| IBIS file imx8qx_21x21_v204.ibs generated by Viper version: 2017.04.12
[IBIS Ver]   6.0
[Comment Char] |_char
[File name]   imx8qxp_21x21_v204.ibs
[File Rev]   2.04
[Date]   Nov 13,2019
[Source]   NXP Viper 2017.04.12
[Notes]
   Warning 'pullup_ref' Exceeds 15 characters: VDD_PCIE_LDO_1P0_CAP was cut to VDD_PCIE_LDO_1P
   Warning 'pullup_ref' Exceeds 15 characters: VDD_PCIE_DIG_1P8_3P3 was cut to VDD_PCIE_DIG_1P
   Warning 'pullup_ref' Exceeds 15 characters: VDD_USB_SS3_LDO_1P0_CAP was cut to VDD_USB_SS3_LDO
   Warning 'pullup_ref' Exceeds 15 characters: VDD_EMMC0_1P8_3P3 was cut to VDD_EMMC0_1P8_3
   Warning 'pullup_ref' Exceeds 15 characters: VDD_EMMC0_VSELECT_1P8_3P3 was cut to VDD_EMMC0_VSELE
   Warning 'pullup_ref' Exceeds 15 characters: VDD_USDHC1_VSELECT_1P8_3P3 was cut to VDD_USDHC1_VSEL
   Warning 'pullup_ref' Exceeds 15 characters: VDD_USDHC1_1P8_3P3 was cut to VDD_USDHC1_1P8_
   Warning 'pullup_ref' Exceeds 15 characters: VDD_ENET0_VSELECT_1P8_2P5_3P3 was cut to VDD_ENET0_VSELE
   Warning 'pullup_ref' Exceeds 15 characters: VDD_ENET0_1P8_2P5_3P3 was cut to VDD_ENET0_1P8_2
   Warning 'pullup_ref' Exceeds 15 characters: VDD_ENET_MDIO_1P8_3P3 was cut to VDD_ENET_MDIO_1
   Warning 'pullup_ref' Exceeds 15 characters: VDD_ESAI_SPDIF_1P8_2P5_3P3 was cut to VDD_ESAI_SPDIF_
   Warning 'pullup_ref' Exceeds 15 characters: VDD_SPI_MCLK_UART_1P8_3P3 was cut to VDD_SPI_MCLK_UA
   Warning 'pullup_ref' Exceeds 15 characters: PCIE0_PHY_PLL_REF_RETURN was cut to PCIE0_PHY_PLL_R
   Warning 'pullup_ref' Exceeds 15 characters: VDD_SPI_SAI_1P8_3P3 was cut to VDD_SPI_SAI_1P8
   Warning 'pullup_ref' Exceeds 15 characters: VDD_PCIE_LDO_1P0_CAP was cut to VDD_PCIE_LDO_1P
   Warning 'pullup_ref' Exceeds 15 characters: VDD_CAN_UART_1P8_3P3 was cut to VDD_CAN_UART_1P
   Warning 'pullup_ref' Exceeds 15 characters: VDD_MIPI_DSI_DIG_1P8_3P3 was cut to VDD_MIPI_DSI_DI
   Warning 'pullup_ref' Exceeds 15 characters: VDD_TMPR_CSI_1P8_3P3 was cut to VDD_TMPR_CSI_1P
   Warning 'pullup_ref' Exceeds 15 characters: VDD_QSPI0B_1P8_3P3 was cut to VDD_QSPI0B_1P8_
   Warning 'pulldown_ref' Exceeds 15 characters: VDD_MIPI_CSI_DIG_1P8 was cut to  VDD_MIPI_CSI_DI
   Warning 'pullup_ref' Exceeds 15 characters: VDD_QSPI0A_1P8_3P3 was cut to VDD_QSPI0A_1P8_
   Warning 'pulldown_ref' Exceeds 15 characters: VDD_SNVS_LDO_1P8_CAP was cut to VDD_SNVS_LDO_1P
[Disclaimer] IMPORTANT NOTICE
  This information is provided on an AS IS basis and without warranty.
  IN NO EVENT SHALL NXP BE LIABLE FOR INCIDENTAL OR CONSEQUENTIAL
  DAMAGES ARISING FROM USE OF THIS INFORMATION. THIS DISCLAIMER OF
  WARRANTY EXTENDS TO THE USER OF THE INFORMATION, AND TO THEIR CUSTOMERS
  OR USERS OF PRODUCTS  AND IS IN LIEU OF ALL WARRANTIES WHETHER EXPRESS,
  IMPLIED, OR STATUTORY, INCLUDING IMPLIED WARRANTIES OF MERCHANTABILITY
  OR FITNESS FOR PARTICULAR PURPOSE.
  NXP does not represent or warrant that the information furnished
  hereunder is free of infringement of any third party patents,
  copyrights, trade secrets, or other intellectual property rights.
  NXP does not represent or warrant that the information is free of
  defect, or that it meets any particular standard, requirements or need
  of the user of the infomation or their customers.
  NXP reserves the right to change the information in this file
  without notice.
   http://www.nxp.com
[Copyright]   (C) Copyright NXP 2006 - 2019, All Rights Reserved.
|   imx8qxp_21x21
[Component] imx8qxp_21x21_v204
[Manufacturer] NXP
[Package]
|   typ   min   max
R_pkg   0.40366   0.037637   0.82546
L_pkg   2.483e-9   4.73e-10   4.759e-9
C_pkg   1.224e-12   7.498e-13   3.887e-12
[Pin]   Signal_name   model_name   R_pin   L_pin   C_pin
AA15   VDD_A35   POWER   0.00219   4.708e-11   1.478e-11
AA17   VDD_A35   POWER   0.00219   4.708e-11   1.478e-11
AA19   VDD_A35   POWER   0.00219   4.708e-11   1.478e-11
AB16   VDD_A35   POWER   0.00219   4.708e-11   1.478e-11
AB18   VDD_A35   POWER   0.00219   4.708e-11   1.478e-11
AB20   VDD_A35   POWER   0.00219   4.708e-11   1.478e-11
V28   VDD_ADC_1P8   POWER   0.04684   4.968e-10   1.587e-12
W25   VDD_ADC_DIG_1P8   POWER   0.02408   3.35e-10   7.513e-13
M14   VDD_ANA0_1P8   POWER   0.02045   2.873e-10   3.689e-12
AB24   VDD_ANA1_1P8   POWER   0.01003   1.805e-10   3.242e-12
Y24   VDD_CAN_UART_1P8_3P3   POWER   0.02207   3.294e-10   7.089e-13
AE23   VDD_CSI_1P8_3P3   POWER   0.0291   4.307e-10   1.073e-12
AC9   VDD_DDR_PLL_1P8   POWER   0.03235   4.677e-10   3.486e-12
AA9   VDD_DDR_VDDQ   POWER   0.00256   3.19e-11   2.867e-11
AA11   VDD_DDR_VDDQ   POWER   0.00256   3.19e-11   2.867e-11
AC11   VDD_DDR_VDDQ   POWER   0.00256   3.19e-11   2.867e-11
AD12   VDD_DDR_VDDQ   POWER   0.00256   3.19e-11   2.867e-11
AE11   VDD_DDR_VDDQ   POWER   0.00256   3.19e-11   2.867e-11
M12   VDD_DDR_VDDQ   POWER   0.00256   3.19e-11   2.867e-11
N9   VDD_DDR_VDDQ   POWER   0.00256   3.19e-11   2.867e-11
N11   VDD_DDR_VDDQ   POWER   0.00256   3.19e-11   2.867e-11
R7   VDD_DDR_VDDQ   POWER   0.00256   3.19e-11   2.867e-11
R11   VDD_DDR_VDDQ   POWER   0.00256   3.19e-11   2.867e-11
T12   VDD_DDR_VDDQ   POWER   0.00256   3.19e-11   2.867e-11
U11   VDD_DDR_VDDQ   POWER   0.00256   3.19e-11   2.867e-11
W11   VDD_DDR_VDDQ   POWER   0.00256   3.19e-11   2.867e-11
Y12   VDD_DDR_VDDQ   POWER   0.00256   3.19e-11   2.867e-11
L19   VDD_EMMC0_1P8_3P3   POWER   0.02931   4.406e-10   9.586e-13
M20   VDD_EMMC0_VSELECT_1P8_3P3   POWER   0.0289   4.327e-10   6.925e-13
M24   VDD_ENET0_1P8_2P5_3P3   POWER   0.02439   3.623e-10   7.403e-13
L23   VDD_ENET0_VSELECT_1P8_2P5_3P3   POWER   0.02814   4.601e-10   1.125e-12
L25   VDD_ENET_MDIO_1P8_3P3   POWER   0.0233   3.037e-10   9.528e-13
N25   VDD_ESAI_SPDIF_1P8_2P5_3P3   POWER   0.01663   2.138e-10   1.247e-12
N23   VDD_GPU   POWER   0.00187   3.523e-11   2.181e-11
P20   VDD_GPU   POWER   0.00187   3.523e-11   2.181e-11
P22   VDD_GPU   POWER   0.00187   3.523e-11   2.181e-11
R21   VDD_GPU   POWER   0.00187   3.523e-11   2.181e-11
T22   VDD_GPU   POWER   0.00187   3.523e-11   2.181e-11
U23   VDD_GPU   POWER   0.00187   3.523e-11   2.181e-11
V20   VDD_GPU   POWER   0.00187   3.523e-11   2.181e-11
W21   VDD_GPU   POWER   0.00187   3.523e-11   2.181e-11
AA23   VDD_MAIN   POWER   0.00038   7.636e-12   1.284e-10
AB12   VDD_MAIN   POWER   0.00038   7.636e-12   1.284e-10
AC13   VDD_MAIN   POWER   0.00038   7.636e-12   1.284e-10
AC17   VDD_MAIN   POWER   0.00038   7.636e-12   1.284e-10
AC21   VDD_MAIN   POWER   0.00038   7.636e-12   1.284e-10
AD14   VDD_MAIN   POWER   0.00038   7.636e-12   1.284e-10
AD22   VDD_MAIN   POWER   0.00038   7.636e-12   1.284e-10
N15   VDD_MAIN   POWER   0.00038   7.636e-12   1.284e-10
N19   VDD_MAIN   POWER   0.00038   7.636e-12   1.284e-10
P12   VDD_MAIN   POWER   0.00038   7.636e-12   1.284e-10
P16   VDD_MAIN   POWER   0.00038   7.636e-12   1.284e-10
P24   VDD_MAIN   POWER   0.00038   7.636e-12   1.284e-10
R13   VDD_MAIN   POWER   0.00038   7.636e-12   1.284e-10
R17   VDD_MAIN   POWER   0.00038   7.636e-12   1.284e-10
T14   VDD_MAIN   POWER   0.00038   7.636e-12   1.284e-10
T18   VDD_MAIN   POWER   0.00038   7.636e-12   1.284e-10
U15   VDD_MAIN   POWER   0.00038   7.636e-12   1.284e-10
U19   VDD_MAIN   POWER   0.00038   7.636e-12   1.284e-10
V12   VDD_MAIN   POWER   0.00038   7.636e-12   1.284e-10
V16   VDD_MAIN   POWER   0.00038   7.636e-12   1.284e-10
V24   VDD_MAIN   POWER   0.00038   7.636e-12   1.284e-10
W13   VDD_MAIN   POWER   0.00038   7.636e-12   1.284e-10
W17   VDD_MAIN   POWER   0.00038   7.636e-12   1.284e-10
Y14   VDD_MAIN   POWER   0.00038   7.636e-12   1.284e-10
Y18   VDD_MAIN   POWER   0.00038   7.636e-12   1.284e-10
Y22   VDD_MAIN   POWER   0.00038   7.636e-12   1.284e-10
AD18   VDD_MIPI_1P0   POWER   0.00784   1.178e-10   4.481e-12
AE19   VDD_MIPI_1P0   POWER   0.00784   1.178e-10   4.481e-12
AD16   VDD_MIPI_1P8   POWER   0.00846   1.296e-10   3.255e-12
AE17   VDD_MIPI_1P8   POWER   0.00846   1.296e-10   3.255e-12
AE21   VDD_MIPI_CSI_DIG_1P8   POWER   0.02051   3.356e-10   8.748e-13
AA25   VDD_MIPI_DSI_DIG_1P8_3P3   POWER   0.0223   3.942e-10   7.725e-13
G13   VDD_PCIE_1P8   POWER   0.05261   4.939e-10   2.52e-12
L11   VDD_PCIE_DIG_1P8_3P3   POWER   0.02609   3.742e-10   9.301e-13
L13   VDD_PCIE_LDO_1P0_CAP   POWER   0.02621   2.855e-10   1.291e-12
AE15   VDD_QSPI0A_1P8_3P3   POWER   0.02715   4.596e-10   9.514e-13
AE13   VDD_QSPI0B_1P8_3P3   POWER   0.02591   4.435e-10   9.193e-13
AC25   VDD_SNVS_4P2   POWER   0.04094   4.39e-10   1.24e-12
AE25   VDD_SNVS_LDO_1P8_CAP   POWER   0.02861   4.218e-10   9.798e-13
R25   VDD_SPI_MCLK_UART_1P8_3P3   POWER   0.02101   3.863e-10   9.493e-13
U25   VDD_SPI_SAI_1P8_3P3   POWER   0.01791   3.169e-10   1.118e-12
AD24   VDD_TMPR_CSI_1P8_3P3   POWER   0.02854   4.826e-10   6.671e-13
M18   VDD_USB_1P8   POWER   0.01867   2.529e-10   1.459e-12
L15   VDD_USB_3P3   POWER   0.01456   2.231e-10   2.366e-12
L17   VDD_USB_OTG_1P0   POWER   0.02825   3.838e-10   7.015e-13
M16   VDD_USB_SS3_LDO_1P0_CAP   POWER   0.02218   3.197e-10   1.184e-12
M22   VDD_USDHC1_1P8_3P3   POWER   0.02734   4.514e-10   8.749e-13
L21   VDD_USDHC1_VSELECT_1P8_3P3   POWER   0.02938   4.213e-10   8.418e-13
U35   ADC_IN0   CSF_1V8_FCGPIO   0.42651   2.631e-9   1.261e-12
U33   ADC_IN1   CSF_1V8_FCGPIO   0.36525   2.261e-9   1.117e-12
V32   ADC_IN2   CSF_1V8_FCGPIO   0.31185   1.955e-9   1.06e-12
V30   ADC_IN3   CSF_1V8_FCGPIO   0.27174   1.778e-9   9.234e-13
W29   ADC_IN4   CSF_1V8_FCGPIO   0.22361   1.51e-9   9.133e-13
V34   ADC_IN5   CSF_1V8_FCGPIO   0.38226   2.352e-9   1.137e-12
U29   ADC_VREFH   POWER   0.16541   1.336e-9   1.06e-12
U31   ADC_VREFL   GND   0.16331   1.278e-9   1.113e-12
AK34   ANA_TEST_OUT_N   NC   0.55674   3.419e-9   1.479e-12
AL35   ANA_TEST_OUT_P   NC   0.55489   3.454e-9   1.49e-12
AK28   CSI_D00   IO_20UM_RES_ANAF   0.30952   1.939e-9   1.008e-12
AL29   CSI_D01   IO_20UM_RES_ANAF   0.37926   2.374e-9   1.138e-12
AP30   CSI_D02   IO_20UM_RES_ANAF   0.50676   3.048e-9   1.397e-12
AJ27   CSI_D03   IO_20UM_RES_ANAF   0.26395   1.704e-9   9.425e-13
AN29   CSI_D04   IO_20UM_RES_ANAF   0.44676   2.71e-9   1.306e-12
AM30   CSI_D05   IO_20UM_RES_ANAF   0.49033   2.894e-9   1.387e-12
AJ25   CSI_D06   IO_20UM_RES_ANAF   0.23567   1.526e-9   9.239e-13
AM28   CSI_D07   IO_20UM_RES_ANAF   0.44578   2.645e-9   1.28e-12
AP28   CSI_EN   3V3SF_1V8_3V3_FCGPIO   0.51053   3.054e-9   1.418e-12
AR29   CSI_HSYNC   IO_20UM_RES_ANAF   0.50745   3.087e-9   1.399e-12
AM26   CSI_MCLK   3V3SF_1V8_3V3_FCGPIO   0.3713   2.281e-9   1.19e-12
AK26   CSI_PCLK   3V3SF_1V8_3V3_FCGPIO   0.32277   2.042e-9   1.037e-12
AR27   CSI_RESET   3V3SF_1V8_3V3_FCGPIO   0.48863   3.001e-9   1.374e-12
AL27   CSI_VSYNC   IO_20UM_RES_ANAF   0.36588   2.261e-9   1.126e-12
AB8   DDR_ATO   NC   0.34374   2.177e-9   9.917e-13
Y6   DDR_CK0_N   PCK_PAD   0.32055   2.016e-9   1.025e-12
W5   DDR_CK0_P   PCK_PAD   0.30751   1.935e-9   1.05e-12
N5   DDR_CK1_N   PCK_PAD   0.34912   2.078e-9   1.033e-12
P6   DDR_CK1_P   PCK_PAD   0.3404   2.05e-9   1.067e-12
W1   DDR_DCF00   PCKE_PAD   0.4081   2.466e-9   1.201e-12
U3   DDR_DCF01   PCKE_PAD   0.39573   2.365e-9   1.079e-12
U1   DDR_DCF03   PCKE_PAD   0.41209   2.476e-9   1.189e-12
U7   DDR_DCF04   PCKE_PAD   0.26915   1.653e-9   8.978e-13
U5   DDR_DCF05   PCKE_PAD   0.28802   1.762e-9   9.477e-13
T2   DDR_DCF07   PCKE_PAD   0.38159   2.286e-9   1.123e-12
AB4   DDR_DCF08   PCKE_PAD   0.33535   2.032e-9   1.075e-12
AB6   DDR_DCF09   PCKE_PAD   0.31122   1.881e-9   1.054e-12
AC5   DDR_DCF10   PCKE_PAD   0.42271   2.539e-9   1.134e-12
W3   DDR_DCF11   PCKE_PAD   0.39581   2.382e-9   1.165e-12
Y8   DDR_DCF12   PCKE_PAD   0.26258   1.59e-9   8.647e-13
Y2   DDR_DCF14   PCKE_PAD   0.43988   2.601e-9   1.26e-12
Y4   DDR_DCF15   PCKE_PAD   0.39283   2.343e-9   1.098e-12
W7   DDR_DCF16   PCKE_PAD   0.22506   1.423e-9   8.936e-13
N3   DDR_DCF17   PCKE_PAD   0.40043   2.368e-9   1.158e-12
L1   DDR_DCF18   PCKE_PAD   0.54939   3.23e-9   1.358e-12
N1   DDR_DCF19   PCKE_PAD   0.47195   2.811e-9   1.296e-12
P4   DDR_DCF20   PCKE_PAD   0.38159   2.233e-9   1.089e-12
T8   DDR_DCF21   PCKE_PAD   0.22786   1.416e-9   8.827e-13
P2   DDR_DCF22   PCKE_PAD   0.44786   2.591e-9   1.196e-12
T4   DDR_DCF23   PCKE_PAD   0.30475   1.872e-9   1.03e-12
T6   DDR_DCF24   PCKE_PAD   0.30086   1.802e-9   9.477e-13
K8   DDR_DCF25   PCKE_PAD   0.37204   2.249e-9   1.113e-12
L7   DDR_DCF26   PCKE_PAD   0.31491   2.008e-9   9.604e-13
K4   DDR_DCF27   PCKE_PAD   0.412   2.421e-9   1.164e-12
K6   DDR_DCF28   PCKE_PAD   0.39245   2.305e-9   1.103e-12
K2   DDR_DCF29   PCKE_PAD   0.46305   2.734e-9   1.263e-12
N7   DDR_DCF30   PCKE_PAD   0.21434   1.379e-9   8.174e-13
L5   DDR_DCF31   PCKE_PAD   0.42725   2.616e-9   1.143e-12
L3   DDR_DCF32   PCKE_PAD   0.41678   2.499e-9   1.169e-12
P8   DDR_DCF33   PCKE_PAD   0.18645   1.263e-9   7.498e-13
AJ7   DDR_DM0   PDDRIO_PAD   0.38383   2.275e-9   1.142e-12
AF4   DDR_DM1   PDDRIO_PAD   0.40315   2.392e-9   1.179e-12
D4   DDR_DM2   PDDRIO_PAD   0.53266   3.078e-9   1.418e-12
E1   DDR_DM3   PDDRIO_PAD   0.74086   4.27e-9   1.815e-12
AP6   DDR_DM4   PDDRIO_PAD   0.48564   2.866e-9   1.328e-12
AF6   DDR_DQ00   PDDRIO_PAD   0.34789   2.063e-9   9.964e-13
AE5   DDR_DQ01   PDDRIO_PAD   0.30627   1.861e-9   1.026e-12
AH8   DDR_DQ02   PDDRIO_PAD   0.38806   2.264e-9   1.109e-12
AF8   DDR_DQ03   PDDRIO_PAD   0.30103   1.788e-9   1.013e-12
AM4   DDR_DQ04   PDDRIO_PAD   0.53729   3.098e-9   1.447e-12
AM6   DDR_DQ05   PDDRIO_PAD   0.55824   3.2e-9   1.443e-12
AL5   DDR_DQ06   PDDRIO_PAD   0.47532   2.794e-9   1.344e-12
AL7   DDR_DQ07   PDDRIO_PAD   0.50156   2.927e-9   1.333e-12
AJ1   DDR_DQ08   PDDRIO_PAD   0.55986   3.265e-9   1.485e-12
AJ3   DDR_DQ09   PDDRIO_PAD   0.51931   2.978e-9   1.364e-12
AH2   DDR_DQ10   PDDRIO_PAD   0.52291   3.031e-9   1.394e-12
AH4   DDR_DQ11   PDDRIO_PAD   0.48438   2.816e-9   1.311e-12
AC3   DDR_DQ12   PDDRIO_PAD   0.39385   2.334e-9   1.15e-12
AE3   DDR_DQ13   PDDRIO_PAD   0.44737   2.593e-9   1.227e-12
AB2   DDR_DQ14   PDDRIO_PAD   0.43448   2.589e-9   1.216e-12
AC1   DDR_DQ15   PDDRIO_PAD   0.50595   3.028e-9   1.287e-12
B6   DDR_DQ16   PDDRIO_PAD   0.60749   3.574e-9   1.522e-12
E9   DDR_DQ17   PDDRIO_PAD   0.50742   3.111e-9   1.313e-12
E7   DDR_DQ18   PDDRIO_PAD   0.4559   2.689e-9   1.295e-12
D8   DDR_DQ19   PDDRIO_PAD   0.54325   3.262e-9   1.355e-12
G7   DDR_DQ20   PDDRIO_PAD   0.46743   2.712e-9   1.304e-12
H8   DDR_DQ21   PDDRIO_PAD   0.50906   2.936e-9   1.288e-12
H6   DDR_DQ22   PDDRIO_PAD   0.4057   2.436e-9   1.192e-12
G5   DDR_DQ23   PDDRIO_PAD   0.45898   2.662e-9   1.251e-12
H2   DDR_DQ24   PDDRIO_PAD   0.77451   4.461e-9   1.879e-12
H4   DDR_DQ25   PDDRIO_PAD   0.7738   4.561e-9   1.785e-12
G3   DDR_DQ26   PDDRIO_PAD   0.73029   4.212e-9   1.787e-12
G1   DDR_DQ27   PDDRIO_PAD   0.82546   4.759e-9   1.895e-12
A7   DDR_DQ28   PDDRIO_PAD   0.5151   3.062e-9   1.35e-12
B4   DDR_DQ29   PDDRIO_PAD   0.58541   3.377e-9   1.536e-12
B2   DDR_DQ30   PDDRIO_PAD   0.64864   3.755e-9   1.64e-12
A5   DDR_DQ31   PDDRIO_PAD   0.55394   3.304e-9   1.492e-12
AL1   DDR_DQ32   PDDRIO_PAD   0.69902   3.996e-9   1.723e-12
AM2   DDR_DQ33   PDDRIO_PAD   0.68978   3.899e-9   1.65e-12
AL3   DDR_DQ34   PDDRIO_PAD   0.60728   3.501e-9   1.582e-12
AP2   DDR_DQ35   PDDRIO_PAD   0.73516   4.145e-9   1.724e-12
AP8   DDR_DQ36   PDDRIO_PAD   0.45415   2.678e-9   1.278e-12
AP10   DDR_DQ37   PDDRIO_PAD   0.49344   2.899e-9   1.314e-12
AR9   DDR_DQ38   PDDRIO_PAD   0.50308   2.973e-9   1.338e-12
AR7   DDR_DQ39   PDDRIO_PAD   0.48449   2.912e-9   1.388e-12
AH6   DDR_DQS0_N   PDQS_PAD   0.47602   2.752e-9   1.322e-12
AJ5   DDR_DQS0_P   PDQS_PAD   0.48689   2.789e-9   1.302e-12
AE1   DDR_DQS1_N   PDQS_PAD   0.53539   3.09e-9   1.4e-12
AF2   DDR_DQS1_P   PDQS_PAD   0.52472   3.013e-9   1.398e-12
E5   DDR_DQS2_N   PDQS_PAD   0.54029   3.111e-9   1.395e-12
D6   DDR_DQS2_P   PDQS_PAD   0.54822   3.239e-9   1.375e-12
E3   DDR_DQS3_N   PDQS_PAD   0.75887   4.285e-9   1.793e-12
D2   DDR_DQS3_P   PDQS_PAD   0.74586   4.218e-9   1.843e-12
AR5   DDR_DQS4_N   PDQS_PAD   0.62598   3.596e-9   1.508e-12
AP4   DDR_DQS4_P   PDQS_PAD   0.61626   3.503e-9   1.593e-12
AC7   DDR_DTO0   PDDRIO_PAD   0.37637   2.321e-9   1.141e-12
AE7   DDR_DTO1   PDDRIO_PAD   0.40575   2.477e-9   1.172e-12
AD8   DDR_VREF   POWER   0.037637   4.73e-10   3.887e-12
G9   DDR_ZQ   NC   0.47928   3.163e-9   2.009e-12
G19   EMMC0_CLK   3V3SF_1V8_3V3_FCGPIO   0.24299   1.577e-9   9.178e-13
D20   EMMC0_CMD   3V3SF_1V8_3V3_FCGPIO   0.35749   2.183e-9   1.114e-12
C21   EMMC0_DATA0   3V3SF_1V8_3V3_FCGPIO   0.40233   2.452e-9   1.222e-12
A21   EMMC0_DATA1   3V3SF_1V8_3V3_FCGPIO   0.43389   2.669e-9   1.273e-12
E21   EMMC0_DATA2   3V3SF_1V8_3V3_FCGPIO   0.34577   2.14e-9   1.047e-12
H20   EMMC0_DATA3   3V3SF_1V8_3V3_FCGPIO   0.19693   1.326e-9   8.274e-13
B22   EMMC0_DATA4   3V3SF_1V8_3V3_FCGPIO   0.40922   2.519e-9   1.201e-12
G21   EMMC0_DATA5   3V3SF_1V8_3V3_FCGPIO   0.2411   1.561e-9   8.981e-13
A23   EMMC0_DATA6   3V3SF_1V8_3V3_FCGPIO   0.47648   2.905e-9   1.346e-12
D22   EMMC0_DATA7   3V3SF_1V8_3V3_FCGPIO   0.38392   2.379e-9   1.207e-12
H22   EMMC0_RESET_B   3V3SF_1V8_3V3_FCGPIO   0.2085   1.381e-9   8.717e-13
F22   EMMC0_STROBE   3V3SF_1V8_3V3_FCGPIO   0.27801   1.763e-9   9.676e-13
D30   ENET0_MDC   3V3SF_1V8_3V3_FCGPIO   0.35839   2.254e-9   1.196e-12
B32   ENET0_MDIO   3V3SF_1V8_3V3_FCGPIO   0.47882   2.938e-9   1.4e-12
F28   ENET0_REFCLK_125M_25M   3V3SF_1V8_3V3_FCGPIO   0.29671   1.976e-9   1.042e-12
D28   ENET0_RGMII_RXC   RGMIIRX_GPIO   0.34785   2.197e-9   1.166e-12
A31   ENET0_RGMII_RXD0   RGMIIRX_GPIO   0.51375   3.163e-9   1.419e-12
C29   ENET0_RGMII_RXD1   RGMIIRX_GPIO   0.42687   2.638e-9   1.308e-12
G27   ENET0_RGMII_RXD2   RGMIIRX_GPIO   0.26051   1.789e-9   9.619e-13
H26   ENET0_RGMII_RXD3   RGMIIRX_GPIO   0.22422   1.541e-9   9.198e-13
B30   ENET0_RGMII_RX_CTL   RGMIIRX_GPIO   0.48399   3.024e-9   1.372e-12
H24   ENET0_RGMII_TXC   RGMIITX_GPIO   0.24969   1.649e-9   9.326e-13
G25   ENET0_RGMII_TXD0   RGMIITX_GPIO   0.25954   1.719e-9   9.815e-13
B28   ENET0_RGMII_TXD1   RGMIITX_GPIO   0.47751   2.912e-9   1.396e-12
E27   ENET0_RGMII_TXD2   RGMIITX_GPIO   0.32018   2.051e-9   1.1e-12
F26   ENET0_RGMII_TXD3   RGMIITX_GPIO   0.27647   1.816e-9   1.02e-12
A29   ENET0_RGMII_TX_CTL   RGMIITX_GPIO   0.52202   3.211e-9   1.493e-12
F30   ESAI0_FSR   RGMIITX_GPIO   0.39537   2.424e-9   1.193e-12
G29   ESAI0_FST   RGMIITX_GPIO   0.29458   1.849e-9   1.035e-12
H28   ESAI0_SCKR   RGMIITX_GPIO   0.28835   1.88e-9   9.652e-13
E31   ESAI0_SCKT   RGMIITX_GPIO   0.42951   2.579e-9   1.293e-12
D32   ESAI0_TX0   RGMIIRX_GPIO   0.5198   3.07e-9   1.429e-12
B34   ESAI0_TX1   RGMIIRX_GPIO   0.60233   3.515e-9   1.568e-12
K28   ESAI0_TX2_RX3   RGMIIRX_GPIO   0.23591   1.548e-9   9.045e-13
C33   ESAI0_TX3_RX2   RGMIIRX_GPIO   0.5599   3.292e-9   1.515e-12
F32   ESAI0_TX4_RX1   RGMIITX_GPIO   0.45945   2.754e-9   1.313e-12
J29   ESAI0_TX5_RX0   RGMIITX_GPIO   0.27518   1.75e-9   9.731e-13
Y34   FLEXCAN0_RX   3V3SF_1V8_3V3_FCGPIO   0.35762   2.213e-9   1.151e-12
Y32   FLEXCAN0_TX   3V3SF_1V8_3V3_FCGPIO   0.30614   1.932e-9   1.019e-12
AA33   FLEXCAN1_RX   3V3SF_1V8_3V3_FCGPIO   0.354   2.21e-9   1.127e-12
AA35   FLEXCAN1_TX   3V3SF_1V8_3V3_FCGPIO   0.40774   2.539e-9   1.249e-12
AB34   FLEXCAN2_RX   3V3SF_1V8_3V3_FCGPIO   0.40111   2.512e-9   1.179e-12
AA31   FLEXCAN2_TX   3V3SF_1V8_3V3_FCGPIO   0.30369   1.932e-9   1.065e-12
AE31   JTAG_TCK   CSF_1V8_FCGPIO   0.31701   2.002e-9   1.07e-12
AH34   JTAG_TDI   CSF_1V8_FCGPIO   0.46348   2.803e-9   1.317e-12
AF32   JTAG_TDO   CSF_1V8_FCGPIO   0.35968   2.233e-9   1.165e-12
AG35   JTAG_TMS   CSF_1V8_FCGPIO   0.48605   2.989e-9   1.367e-12
AD28   JTAG_TRST_B   CSF_1V8_FCGPIO   0.19606   1.354e-9   8.282e-13
G35   MCLK_IN0   3V3SF_1V8_3V3_FCGPIO   0.55731   3.374e-9   1.518e-12
M28   MCLK_IN1   3V3SF_1V8_3V3_FCGPIO   0.20261   1.389e-9   8.304e-13
L29   MCLK_OUT0   3V3SF_1V8_3V3_FCGPIO   0.32644   2.033e-9   1.062e-12
AN21   MIPI_CSI0_CLK_N   MIPI_CSI   0.49498   3.004e-9   1.369e-12
AR21   MIPI_CSI0_CLK_P   MIPI_CSI   0.48962   3.061e-9   1.357e-12
AM22   MIPI_CSI0_DATA0_N   MIPI_CSI   0.49701   2.96e-9   1.377e-12
AP22   MIPI_CSI0_DATA0_P   MIPI_CSI   0.49255   3.041e-9   1.353e-12
AM20   MIPI_CSI0_DATA1_N   MIPI_CSI   0.48506   2.903e-9   1.34e-12
AP20   MIPI_CSI0_DATA1_P   MIPI_CSI   0.48156   2.988e-9   1.341e-12
AN23   MIPI_CSI0_DATA2_N   MIPI_CSI   0.47971   2.928e-9   1.33e-12
AR23   MIPI_CSI0_DATA2_P   MIPI_CSI   0.47871   3.004e-9   1.318e-12
AN19   MIPI_CSI0_DATA3_N   MIPI_CSI   0.50138   3.041e-9   1.391e-12
AR19   MIPI_CSI0_DATA3_P   MIPI_CSI   0.49818   3.108e-9   1.377e-12
AR25   MIPI_CSI0_GPIO0_00   CSF_1V8_FCGPIO   0.49968   3.044e-9   1.364e-12
AP24   MIPI_CSI0_GPIO0_01   CSF_1V8_FCGPIO   0.45119   2.799e-9   1.3e-12
AP26   MIPI_CSI0_I2C0_SCL   CSF_1V8_FCGPIO   0.46856   2.831e-9   1.317e-12
AM24   MIPI_CSI0_I2C0_SDA   CSF_1V8_FCGPIO   0.37935   2.333e-9   1.161e-12
AN25   MIPI_CSI0_MCLK_OUT   CSF_1V8_FCGPIO   0.4119   2.52e-9   1.23e-12
AJ19   MIPI_DSI0_CLK_N   MIPI_LVDS_DSI   0.42988   2.6e-9   1.28e-12
AK20   MIPI_DSI0_CLK_P   MIPI_LVDS_DSI   0.43   2.588e-9   1.28e-12
AJ21   MIPI_DSI0_DATA0_N   MIPI_LVDS_DSI   0.44241   2.691e-9   1.272e-12
AK22   MIPI_DSI0_DATA0_P   MIPI_LVDS_DSI   0.43697   2.659e-9   1.291e-12
AJ17   MIPI_DSI0_DATA1_N   MIPI_LVDS_DSI   0.446   2.684e-9   1.3e-12
AK18   MIPI_DSI0_DATA1_P   MIPI_LVDS_DSI   0.44294   2.68e-9   1.263e-12
AJ23   MIPI_DSI0_DATA2_N   MIPI_LVDS_DSI   0.4275   2.61e-9   1.283e-12
AK24   MIPI_DSI0_DATA2_P   MIPI_LVDS_DSI   0.42483   2.567e-9   1.308e-12
AJ15   MIPI_DSI0_DATA3_N   MIPI_LVDS_DSI   0.4266   2.617e-9   1.321e-12
AK16   MIPI_DSI0_DATA3_P   MIPI_LVDS_DSI   0.42334   2.594e-9   1.304e-12
AD32   MIPI_DSI0_GPIO0_00   3V3SF_1V8_3V3_FCGPIO   0.34528   2.149e-9   1.121e-12
AE35   MIPI_DSI0_GPIO0_01   3V3SF_1V8_3V3_FCGPIO   0.45009   2.81e-9   1.311e-12
AC31   MIPI_DSI0_I2C0_SCL   3V3SF_1V8_3V3_FCGPIO   0.28263   1.842e-9   1.016e-12
AB28   MIPI_DSI0_I2C0_SDA   3V3SF_1V8_3V3_FCGPIO   0.26255   1.741e-9   9.789e-13
AM16   MIPI_DSI1_CLK_N   MIPI_LVDS_DSI   0.44472   2.729e-9   1.272e-12
AP16   MIPI_DSI1_CLK_P   MIPI_LVDS_DSI   0.4479   2.808e-9   1.249e-12
AN15   MIPI_DSI1_DATA0_N   MIPI_LVDS_DSI   0.44235   2.726e-9   1.297e-12
AR15   MIPI_DSI1_DATA0_P   MIPI_LVDS_DSI   0.44312   2.835e-9   1.257e-12
AN17   MIPI_DSI1_DATA1_N   MIPI_LVDS_DSI   0.46315   2.86e-9   1.34e-12
AR17   MIPI_DSI1_DATA1_P   MIPI_LVDS_DSI   0.46309   2.964e-9   1.298e-12
AM14   MIPI_DSI1_DATA2_N   MIPI_LVDS_DSI   0.4465   2.703e-9   1.323e-12
AP14   MIPI_DSI1_DATA2_P   MIPI_LVDS_DSI   0.44932   2.756e-9   1.276e-12
AM18   MIPI_DSI1_DATA3_N   MIPI_LVDS_DSI   0.43264   2.647e-9   1.286e-12
AP18   MIPI_DSI1_DATA3_P   MIPI_LVDS_DSI   0.43548   2.732e-9   1.249e-12
AD30   MIPI_DSI1_GPIO0_00   3V3SF_1V8_3V3_FCGPIO   0.27866   1.821e-9   1.009e-12
AF34   MIPI_DSI1_GPIO0_01   3V3SF_1V8_3V3_FCGPIO   0.46083   2.793e-9   1.315e-12
AE33   MIPI_DSI1_I2C0_SCL   3V3SF_1V8_3V3_FCGPIO   0.39576   2.444e-9   1.182e-12
AC29   MIPI_DSI1_I2C0_SDA   3V3SF_1V8_3V3_FCGPIO   0.2436   1.627e-9   9.374e-13
AH28   ON_OFF_BUTTON   IO_20UM_RES_ANAF_1V8   0.29563   1.902e-9   9.364e-13
G11   PCIE0_PHY_PLL_REF_RETURN   GND   0.054501   6.217e-10   2.107e-12
B12   PCIE0_RX0_N   ABI_SERDES   0.42156   2.861e-9   1.296e-12
A13   PCIE0_RX0_P   ABI_SERDES   0.41663   2.936e-9   1.279e-12
A9   PCIE0_TX0_N   ABI_SERDES   0.40731   2.81e-9   1.245e-12
B10   PCIE0_TX0_P   ABI_SERDES   0.40375   2.848e-9   1.233e-12
D10   PCIE_CTRL0_CLKREQ_B   3V3SF_1V8_3V3_FCGPIO   0.40135   2.53e-9   1.265e-12
H10   PCIE_CTRL0_PERST_B   3V3SF_1V8_3V3_FCGPIO   0.12512   9.972e-10   7.745e-13
A11   PCIE_CTRL0_WAKE_B   3V3SF_1V8_3V3_FCGPIO   0.47936   3.039e-9   1.422e-12
D12   PCIE_REFCLK100M_N   PCIEREFCLKIO_N   0.32667   2.067e-9   1.106e-12
E11   PCIE_REFCLK100M_P   PCIEREFCLKIO_P   0.32662   2.076e-9   1.105e-12
F12   PCIE_REF_QR   NC   0.28819   1.902e-9   9.99e-13
H12   PCIE_REXT   NC   0.24788   1.989e-9   1.229e-12
AJ35   PMIC_I2C_SCL   CSF_1V8_FCGPIO   0.50002   3.076e-9   1.421e-12
AH32   PMIC_I2C_SDA   CSF_1V8_FCGPIO   0.42322   2.576e-9   1.277e-12
AJ33   PMIC_INT_B   CSF_1V8_FCGPIO   0.45318   2.749e-9   1.321e-12
AR31   PMIC_ON_REQ   IO_20UM_RES_ANAF_1V8   0.5575   3.345e-9   1.472e-12
AG31   POR_B   CSF_1V8_FCGPIO   0.34044   2.142e-9   1.115e-12
AK14   QSPI0A_DATA0   3V3SF_1V8_3V3_FCGPIO   0.25143   1.633e-9   9.428e-13
AR13   QSPI0A_DATA1   3V3SF_1V8_3V3_FCGPIO   0.43046   2.722e-9   1.268e-12
AJ13   QSPI0A_DATA2   3V3SF_1V8_3V3_FCGPIO   0.23405   1.502e-9   8.871e-13
AH12   QSPI0A_DATA3   3V3SF_1V8_3V3_FCGPIO   0.19228   1.314e-9   8.523e-13
AL11   QSPI0A_DQS   3V3SF_1V8_3V3_FCGPIO   0.34951   2.174e-9   1.14e-12
AP12   QSPI0A_SCLK   3V3SF_1V8_3V3_FCGPIO   0.49462   2.929e-9   1.344e-12
AM12   QSPI0A_SS0_B   3V3SF_1V8_3V3_FCGPIO   0.351   2.16e-9   1.116e-12
AK12   QSPI0A_SS1_B   3V3SF_1V8_3V3_FCGPIO   0.3075   1.925e-9   1.051e-12
AM10   QSPI0B_DATA0   3V3SF_1V8_3V3_FCGPIO   0.37156   2.27e-9   1.152e-12
AL9   QSPI0B_DATA1   3V3SF_1V8_3V3_FCGPIO   0.38652   2.345e-9   1.16e-12
AJ11   QSPI0B_DATA2   3V3SF_1V8_3V3_FCGPIO   0.22484   1.496e-9   8.868e-13
AM8   QSPI0B_DATA3   3V3SF_1V8_3V3_FCGPIO   0.40193   2.44e-9   1.234e-12
AK10   QSPI0B_DQS   3V3SF_1V8_3V3_FCGPIO   0.28042   1.81e-9   1.013e-12
AR11   QSPI0B_SCLK   3V3SF_1V8_3V3_FCGPIO   0.48845   2.981e-9   1.356e-12
AH10   QSPI0B_SS0_B   3V3SF_1V8_3V3_FCGPIO   0.19767   1.323e-9   8.385e-13
AJ9   QSPI0B_SS1_B   3V3SF_1V8_3V3_FCGPIO   0.28652   1.795e-9   9.915e-13
AP32   RTC_XTALI   IO_20UM_RES_ANAF_1V8   0.54741   3.327e-9   1.416e-12
AM32   RTC_XTALO   IO_20UM_RES_ANAF_1V8   0.47797   2.858e-9   1.315e-12
M34   SAI0_RXD   3V3SF_1V8_3V3_FCGPIO   0.47628   2.864e-9   1.356e-12
J35   SAI0_TXC   3V3SF_1V8_3V3_FCGPIO   0.51909   3.139e-9   1.421e-12
K34   SAI0_TXD   3V3SF_1V8_3V3_FCGPIO   0.46709   2.828e-9   1.341e-12
L33   SAI0_TXFS   3V3SF_1V8_3V3_FCGPIO   0.41937   2.585e-9   1.245e-12
L35   SAI1_RXC   3V3SF_1V8_3V3_FCGPIO   0.49409   3.028e-9   1.399e-12
M32   SAI1_RXD   3V3SF_1V8_3V3_FCGPIO   0.36595   2.282e-9   1.168e-12
N35   SAI1_RXFS   3V3SF_1V8_3V3_FCGPIO   0.45217   2.811e-9   1.304e-12
AJ31   SCU_BOOT_MODE0   CSF_1V8_FCGPIO   0.37261   2.344e-9   1.178e-12
AK32   SCU_BOOT_MODE1   CSF_1V8_FCGPIO   0.44725   2.738e-9   1.324e-12
AL31   SCU_BOOT_MODE2   CSF_1V8_FCGPIO   0.45121   2.817e-9   1.277e-12
AJ29   SCU_BOOT_MODE3   CSF_1V8_FCGPIO   0.39107   2.552e-9   1.182e-12
AF28   SCU_GPIO0_00   CSF_1V8_FCGPIO   0.26999   1.757e-9   1.001e-12
AH30   SCU_GPIO0_01   CSF_1V8_FCGPIO   0.35006   2.195e-9   1.14e-12
AG29   SCU_PMIC_STANDBY   CSF_1V8_FCGPIO   0.28196   1.838e-9   9.922e-13
E35   SPDIF0_EXT_CLK   RGMIITX_GPIO   0.57126   3.398e-9   1.532e-12
G31   SPDIF0_RX   RGMIIRX_GPIO   0.42747   2.583e-9   1.252e-12
D34   SPDIF0_TX   RGMIIRX_GPIO   0.58257   3.431e-9   1.561e-12
R33   SPI0_CS0   3V3SF_1V8_3V3_FCGPIO   0.37381   2.352e-9   1.172e-12
R35   SPI0_CS1   3V3SF_1V8_3V3_FCGPIO   0.43046   2.673e-9   1.266e-12
P30   SPI0_SCK   3V3SF_1V8_3V3_FCGPIO   0.27879   1.846e-9   9.634e-13
P34   SPI0_SDI   3V3SF_1V8_3V3_FCGPIO   0.40042   2.473e-9   1.203e-12
R31   SPI0_SDO   3V3SF_1V8_3V3_FCGPIO   0.31042   1.967e-9   1.031e-12
P28   SPI2_CS0   3V3SF_1V8_3V3_FCGPIO   0.22697   1.549e-9   8.97e-13
R29   SPI2_SCK   3V3SF_1V8_3V3_FCGPIO   0.22708   1.592e-9   8.776e-13
N31   SPI2_SDI   3V3SF_1V8_3V3_FCGPIO   0.3277   2.118e-9   1.082e-12
P32   SPI2_SDO   3V3SF_1V8_3V3_FCGPIO   0.33999   2.13e-9   1.132e-12
J31   SPI3_CS0   3V3SF_1V8_3V3_FCGPIO   0.39284   2.418e-9   1.194e-12
K30   SPI3_CS1   3V3SF_1V8_3V3_FCGPIO   0.34945   2.169e-9   1.116e-12
H32   SPI3_SCK   3V3SF_1V8_3V3_FCGPIO   0.41524   2.523e-9   1.275e-12
G33   SPI3_SDI   3V3SF_1V8_3V3_FCGPIO   0.51204   3.045e-9   1.416e-12
F34   SPI3_SDO   3V3SF_1V8_3V3_FCGPIO   0.54161   3.213e-9   1.457e-12
AE29   TEST_MODE_SELECT   CSF_1V8_FCGPIO   0.2439   1.621e-9   9.126e-13
AB32   UART0_RX   3V3SF_1V8_3V3_FCGPIO   0.33344   2.087e-9   1.106e-12
AA29   UART0_TX   3V3SF_1V8_3V3_FCGPIO   0.19748   1.391e-9   8.474e-13
K32   UART1_CTS_B   3V3SF_1V8_3V3_FCGPIO   0.41749   2.526e-9   1.258e-12
N29   UART1_RTS_B   3V3SF_1V8_3V3_FCGPIO   0.26313   1.73e-9   9.823e-13
L31   UART1_RX   3V3SF_1V8_3V3_FCGPIO   0.35873   2.234e-9   1.158e-12
H34   UART1_TX   3V3SF_1V8_3V3_FCGPIO   0.51338   3.086e-9   1.439e-12
AD34   UART2_RX   3V3SF_1V8_3V3_FCGPIO   0.42931   2.632e-9   1.262e-12
AC35   UART2_TX   3V3SF_1V8_3V3_FCGPIO   0.43022   2.683e-9   1.274e-12
E19   USB_OTG1_DN   USB_NXP   0.28705   1.992e-9   9.273e-13
D18   USB_OTG1_DP   USB_NXP   0.29599   1.997e-9   9.267e-13
G17   USB_OTG1_ID   NC   0.18553   1.34e-9   8.412e-13
H18   USB_OTG1_VBUS   USB_NXP   0.16468   1.199e-9   8.524e-13
D16   USB_OTG2_DN   USB2_CDN   0.28757   2.012e-9   8.975e-13
E17   USB_OTG2_DP   USB2_CDN   0.28814   2.024e-9   8.979e-13
F16   USB_OTG2_ID   NC   0.25295   1.684e-9   9.881e-13
D14   USB_OTG2_REXT   NC   0.23481   1.751e-9   1.314e-12
H16   USB_OTG2_VBUS   NC   0.19865   1.497e-9   8.131e-13
E13   USB_SS3_REXT   NC   0.2561   2.018e-9   1.268e-12
B18   USB_SS3_RX_N   USB3_RX   0.42832   2.845e-9   1.246e-12
A19   USB_SS3_RX_P   USB3_RX   0.43031   2.852e-9   1.249e-12
F14   USB_SS3_TC0   3V3SF_3V3_FCGPIO   0.24184   1.566e-9   9.365e-13
H14   USB_SS3_TC1   3V3SF_3V3_FCGPIO   0.21355   1.461e-9   8.627e-13
G15   USB_SS3_TC2   3V3SF_3V3_FCGPIO   0.23763   1.667e-9   9.232e-13
C15   USB_SS3_TC3   3V3SF_3V3_FCGPIO   0.35732   2.268e-9   1.138e-12
A15   USB_SS3_TX_N   USB3_TX   0.37617   2.585e-9   1.118e-12
B16   USB_SS3_TX_P   USB3_TX   0.37724   2.508e-9   1.123e-12
E23   USDHC1_CD_B   3V3SF_1V8_3V3_FCGPIO   0.38731   2.428e-9   1.227e-12
G23   USDHC1_CLK   3V3SF_1V8_3V3_FCGPIO   0.21835   1.534e-9   9.013e-13
C25   USDHC1_CMD   3V3SF_1V8_3V3_FCGPIO   0.39976   2.479e-9   1.221e-12
A27   USDHC1_DATA0   3V3SF_1V8_3V3_FCGPIO   0.51753   3.177e-9   1.441e-12
B26   USDHC1_DATA1   3V3SF_1V8_3V3_FCGPIO   0.44612   2.761e-9   1.309e-12
D26   USDHC1_DATA2   3V3SF_1V8_3V3_FCGPIO   0.38746   2.397e-9   1.207e-12
E25   USDHC1_DATA3   3V3SF_1V8_3V3_FCGPIO   0.31816   2.055e-9   1.089e-12
B24   USDHC1_RESET_B   3V3SF_1V8_3V3_FCGPIO   0.49397   3.005e-9   1.385e-12
A25   USDHC1_VSELECT   3V3SF_1V8_3V3_FCGPIO   0.49179   3.025e-9   1.419e-12
D24   USDHC1_WP   3V3SF_1V8_3V3_FCGPIO   0.39297   2.441e-9   1.227e-12
AP34   XTALI   IO_20UM_RES_ANAF_1V8   0.54935   3.26e-9   1.467e-12
AM34   XTALO   IO_20UM_RES_ANAF_1V8   0.48625   2.947e-9   1.386e-12
A3   VSS_MAIN   GND   NA   NA   NA
A17   VSS_MAIN   GND   NA   NA   NA
A33   VSS_MAIN   GND   NA   NA   NA
AA1   VSS_MAIN   GND   NA   NA   NA
AA3   VSS_MAIN   GND   NA   NA   NA
AA5   VSS_MAIN   GND   NA   NA   NA
AA7   VSS_MAIN   GND   NA   NA   NA
AA13   VSS_MAIN   GND   NA   NA   NA
AA21   VSS_MAIN   GND   NA   NA   NA
AA27   VSS_MAIN   GND   NA   NA   NA
AB10   VSS_MAIN   GND   NA   NA   NA
AB14   VSS_MAIN   GND   NA   NA   NA
AB22   VSS_MAIN   GND   NA   NA   NA
AB26   VSS_MAIN   GND   NA   NA   NA
AB30   VSS_MAIN   GND   NA   NA   NA
AC15   VSS_MAIN   GND   NA   NA   NA
AC19   VSS_MAIN   GND   NA   NA   NA
AC23   VSS_MAIN   GND   NA   NA   NA
AC27   VSS_MAIN   GND   NA   NA   NA
AC33   VSS_MAIN   GND   NA   NA   NA
AD2   VSS_MAIN   GND   NA   NA   NA
AD4   VSS_MAIN   GND   NA   NA   NA
AD6   VSS_MAIN   GND   NA   NA   NA
AD10   VSS_MAIN   GND   NA   NA   NA
AD20   VSS_MAIN   GND   NA   NA   NA
AD26   VSS_MAIN   GND   NA   NA   NA
AE9   VSS_MAIN   GND   NA   NA   NA
AE27   VSS_MAIN   GND   NA   NA   NA
AF10   VSS_MAIN   GND   NA   NA   NA
AF12   VSS_MAIN   GND   NA   NA   NA
AF14   VSS_MAIN   GND   NA   NA   NA
AF16   VSS_MAIN   GND   NA   NA   NA
AF18   VSS_MAIN   GND   NA   NA   NA
AF20   VSS_MAIN   GND   NA   NA   NA
AF22   VSS_MAIN   GND   NA   NA   NA
AF24   VSS_MAIN   GND   NA   NA   NA
AF26   VSS_MAIN   GND   NA   NA   NA
AF30   VSS_MAIN   GND   NA   NA   NA
AG1   VSS_MAIN   GND   NA   NA   NA
AG3   VSS_MAIN   GND   NA   NA   NA
AG5   VSS_MAIN   GND   NA   NA   NA
AG7   VSS_MAIN   GND   NA   NA   NA
AG9   VSS_MAIN   GND   NA   NA   NA
AG11   VSS_MAIN   GND   NA   NA   NA
AG13   VSS_MAIN   GND   NA   NA   NA
AG15   VSS_MAIN   GND   NA   NA   NA
AG17   VSS_MAIN   GND   NA   NA   NA
AG19   VSS_MAIN   GND   NA   NA   NA
AG21   VSS_MAIN   GND   NA   NA   NA
AG23   VSS_MAIN   GND   NA   NA   NA
AG25   VSS_MAIN   GND   NA   NA   NA
AG27   VSS_MAIN   GND   NA   NA   NA
AG33   VSS_MAIN   GND   NA   NA   NA
AH14   VSS_MAIN   GND   NA   NA   NA
AH16   VSS_MAIN   GND   NA   NA   NA
AH18   VSS_MAIN   GND   NA   NA   NA
AH20   VSS_MAIN   GND   NA   NA   NA
AH22   VSS_MAIN   GND   NA   NA   NA
AH24   VSS_MAIN   GND   NA   NA   NA
AH26   VSS_MAIN   GND   NA   NA   NA
AK2   VSS_MAIN   GND   NA   NA   NA
AK4   VSS_MAIN   GND   NA   NA   NA
AK6   VSS_MAIN   GND   NA   NA   NA
AK8   VSS_MAIN   GND   NA   NA   NA
AK30   VSS_MAIN   GND   NA   NA   NA
AL13   VSS_MAIN   GND   NA   NA   NA
AL15   VSS_MAIN   GND   NA   NA   NA
AL17   VSS_MAIN   GND   NA   NA   NA
AL19   VSS_MAIN   GND   NA   NA   NA
AL21   VSS_MAIN   GND   NA   NA   NA
AL23   VSS_MAIN   GND   NA   NA   NA
AL25   VSS_MAIN   GND   NA   NA   NA
AL33   VSS_MAIN   GND   NA   NA   NA
AN1   VSS_MAIN   GND   NA   NA   NA
AN3   VSS_MAIN   GND   NA   NA   NA
AN5   VSS_MAIN   GND   NA   NA   NA
AN7   VSS_MAIN   GND   NA   NA   NA
AN9   VSS_MAIN   GND   NA   NA   NA
AN11   VSS_MAIN   GND   NA   NA   NA
AN13   VSS_MAIN   GND   NA   NA   NA
AN27   VSS_MAIN   GND   NA   NA   NA
AN31   VSS_MAIN   GND   NA   NA   NA
AN33   VSS_MAIN   GND   NA   NA   NA
AN35   VSS_MAIN   GND   NA   NA   NA
AR3   VSS_MAIN   GND   NA   NA   NA
AR33   VSS_MAIN   GND   NA   NA   NA
B8   VSS_MAIN   GND   NA   NA   NA
B14   VSS_MAIN   GND   NA   NA   NA
B20   VSS_MAIN   GND   NA   NA   NA
C1   VSS_MAIN   GND   NA   NA   NA
C3   VSS_MAIN   GND   NA   NA   NA
C5   VSS_MAIN   GND   NA   NA   NA
C7   VSS_MAIN   GND   NA   NA   NA
C9   VSS_MAIN   GND   NA   NA   NA
C11   VSS_MAIN   GND   NA   NA   NA
C13   VSS_MAIN   GND   NA   NA   NA
C17   VSS_MAIN   GND   NA   NA   NA
C19   VSS_MAIN   GND   NA   NA   NA
C23   VSS_MAIN   GND   NA   NA   NA
C27   VSS_MAIN   GND   NA   NA   NA
C31   VSS_MAIN   GND   NA   NA   NA
C35   VSS_MAIN   GND   NA   NA   NA
E15   VSS_MAIN   GND   NA   NA   NA
E29   VSS_MAIN   GND   NA   NA   NA
E33   VSS_MAIN   GND   NA   NA   NA
F2   VSS_MAIN   GND   NA   NA   NA
F4   VSS_MAIN   GND   NA   NA   NA
F6   VSS_MAIN   GND   NA   NA   NA
F8   VSS_MAIN   GND   NA   NA   NA
F10   VSS_MAIN   GND   NA   NA   NA
F18   VSS_MAIN   GND   NA   NA   NA
F20   VSS_MAIN   GND   NA   NA   NA
F24   VSS_MAIN   GND   NA   NA   NA
H30   VSS_MAIN   GND   NA   NA   NA
J1   VSS_MAIN   GND   NA   NA   NA
J3   VSS_MAIN   GND   NA   NA   NA
J5   VSS_MAIN   GND   NA   NA   NA
J7   VSS_MAIN   GND   NA   NA   NA
J9   VSS_MAIN   GND   NA   NA   NA
J11   VSS_MAIN   GND   NA   NA   NA
J13   VSS_MAIN   GND   NA   NA   NA
J15   VSS_MAIN   GND   NA   NA   NA
J17   VSS_MAIN   GND   NA   NA   NA
J19   VSS_MAIN   GND   NA   NA   NA
J21   VSS_MAIN   GND   NA   NA   NA
J23   VSS_MAIN   GND   NA   NA   NA
J25   VSS_MAIN   GND   NA   NA   NA
J27   VSS_MAIN   GND   NA   NA   NA
J33   VSS_MAIN   GND   NA   NA   NA
K10   VSS_MAIN   GND   NA   NA   NA
K12   VSS_MAIN   GND   NA   NA   NA
K14   VSS_MAIN   GND   NA   NA   NA
K16   VSS_MAIN   GND   NA   NA   NA
K18   VSS_MAIN   GND   NA   NA   NA
K20   VSS_MAIN   GND   NA   NA   NA
K22   VSS_MAIN   GND   NA   NA   NA
K24   VSS_MAIN   GND   NA   NA   NA
K26   VSS_MAIN   GND   NA   NA   NA
L9   VSS_MAIN   GND   NA   NA   NA
L27   VSS_MAIN   GND   NA   NA   NA
M2   VSS_MAIN   GND   NA   NA   NA
M4   VSS_MAIN   GND   NA   NA   NA
M6   VSS_MAIN   GND   NA   NA   NA
M8   VSS_MAIN   GND   NA   NA   NA
M10   VSS_MAIN   GND   NA   NA   NA
M26   VSS_MAIN   GND   NA   NA   NA
M30   VSS_MAIN   GND   NA   NA   NA
N13   VSS_MAIN   GND   NA   NA   NA
N17   VSS_MAIN   GND   NA   NA   NA
N21   VSS_MAIN   GND   NA   NA   NA
N27   VSS_MAIN   GND   NA   NA   NA
N33   VSS_MAIN   GND   NA   NA   NA
P10   VSS_MAIN   GND   NA   NA   NA
P14   VSS_MAIN   GND   NA   NA   NA
P18   VSS_MAIN   GND   NA   NA   NA
P26   VSS_MAIN   GND   NA   NA   NA
R1   VSS_MAIN   GND   NA   NA   NA
R3   VSS_MAIN   GND   NA   NA   NA
R5   VSS_MAIN   GND   NA   NA   NA
R9   VSS_MAIN   GND   NA   NA   NA
R15   VSS_MAIN   GND   NA   NA   NA
R19   VSS_MAIN   GND   NA   NA   NA
R23   VSS_MAIN   GND   NA   NA   NA
R27   VSS_MAIN   GND   NA   NA   NA
T10   VSS_MAIN   GND   NA   NA   NA
T16   VSS_MAIN   GND   NA   NA   NA
T20   VSS_MAIN   GND   NA   NA   NA
T24   VSS_MAIN   GND   NA   NA   NA
T26   VSS_MAIN   GND   NA   NA   NA
T28   VSS_MAIN   GND   NA   NA   NA
T30   VSS_MAIN   GND   NA   NA   NA
T32   VSS_MAIN   GND   NA   NA   NA
T34   VSS_MAIN   GND   NA   NA   NA
U9   VSS_MAIN   GND   NA   NA   NA
U13   VSS_MAIN   GND   NA   NA   NA
U17   VSS_MAIN   GND   NA   NA   NA
U21   VSS_MAIN   GND   NA   NA   NA
U27   VSS_MAIN   GND   NA   NA   NA
V2   VSS_MAIN   GND   NA   NA   NA
V4   VSS_MAIN   GND   NA   NA   NA
V6   VSS_MAIN   GND   NA   NA   NA
V8   VSS_MAIN   GND   NA   NA   NA
V10   VSS_MAIN   GND   NA   NA   NA
V14   VSS_MAIN   GND   NA   NA   NA
V18   VSS_MAIN   GND   NA   NA   NA
V22   VSS_MAIN   GND   NA   NA   NA
V26   VSS_MAIN   GND   NA   NA   NA
W9   VSS_MAIN   GND   NA   NA   NA
W15   VSS_MAIN   GND   NA   NA   NA
W19   VSS_MAIN   GND   NA   NA   NA
W23   VSS_MAIN   GND   NA   NA   NA
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[Pin Mapping]   pulldown_ref   pullup_ref   gnd_clamp_ref   power_clamp_ref
A3   GND   NC   NC   NC
A5   GND   VDD_DDR_VDDQ   GND   VDD_DDR_VDDQ
A7   GND   VDD_DDR_VDDQ   GND   VDD_DDR_VDDQ
A9   GND   VDD_PCIE_LDO_1P   GND   VDD_PCIE_LDO_1P
A11   GND   VDD_PCIE_DIG_1P   GND   VDD_PCIE_DIG_1P
A13   GND   VDD_PCIE_LDO_1P   GND   VDD_PCIE_LDO_1P
A15   GND   VDD_USB_1P8   GND   VDD_USB_1P8
A17   GND   NC   NC   NC
A19   GND   VDD_USB_1P8   GND   VDD_USB_1P8
A21   GND   VDD_EMMC0_1P8_3   GND   VDD_EMMC0_1P8_3
A23   GND   VDD_EMMC0_VSELE   GND   VDD_EMMC0_VSELE
A25   GND   VDD_USDHC1_VSEL   GND   VDD_USDHC1_VSEL
A27   GND   VDD_USDHC1_1P8_   GND   VDD_USDHC1_1P8_
A29   GND   VDD_ENET0_VSELE   GND   VDD_ENET0_VSELE
A31   GND   VDD_ENET0_1P8_2   GND   VDD_ENET0_1P8_2
A33   GND   NC   NC   NC
B2   GND   VDD_DDR_VDDQ   GND   VDD_DDR_VDDQ
B4   GND   VDD_DDR_VDDQ   GND   VDD_DDR_VDDQ
B6   GND   VDD_DDR_VDDQ   GND   VDD_DDR_VDDQ
B8   GND   NC   NC   NC
B10   GND   VDD_PCIE_LDO_1P   GND   VDD_PCIE_LDO_1P
B12   GND   VDD_PCIE_LDO_1P   GND   VDD_PCIE_LDO_1P
B14   GND   NC   NC   NC
B16   GND   VDD_USB_1P8   GND   VDD_USB_1P8
B18   GND   VDD_USB_1P8   GND   VDD_USB_1P8
B20   GND   NC   NC   NC
B22   GND   VDD_EMMC0_VSELE   GND   VDD_EMMC0_VSELE
B24   GND   VDD_USDHC1_VSEL   GND   VDD_USDHC1_VSEL
B26   GND   VDD_USDHC1_1P8_   GND   VDD_USDHC1_1P8_
B28   GND   VDD_ENET0_VSELE   GND   VDD_ENET0_VSELE
B30   GND   VDD_ENET0_1P8_2   GND   VDD_ENET0_1P8_2
B32   GND   VDD_ENET_MDIO_1   GND   VDD_ENET_MDIO_1
B34   GND   VDD_ESAI_SPDIF_   GND   VDD_ESAI_SPDIF_
C1   GND   NC   NC   NC
C3   GND   NC   NC   NC
C5   GND   NC   NC   NC
C7   GND   NC   NC   NC
C9   GND   NC   NC   NC
C11   GND   NC   NC   NC
C13   GND   NC   NC   NC
C15   GND   VDD_USB_3P3   GND   VDD_USB_3P3
C17   GND   NC   NC   NC
C19   GND   NC   NC   NC
C21   GND   VDD_EMMC0_1P8_3   GND   VDD_EMMC0_1P8_3
C23   GND   NC   NC   NC
C25   GND   VDD_USDHC1_1P8_   GND   VDD_USDHC1_1P8_
C27   GND   NC   NC   NC
C29   GND   VDD_ENET0_1P8_2   GND   VDD_ENET0_1P8_2
C31   GND   NC   NC   NC
C33   GND   VDD_ESAI_SPDIF_   GND   VDD_ESAI_SPDIF_
C35   GND   NC   NC   NC
D2   GND   VDD_DDR_VDDQ   GND   VDD_DDR_VDDQ
D4   GND   VDD_DDR_VDDQ   GND   VDD_DDR_VDDQ
D6   GND   VDD_DDR_VDDQ   GND   VDD_DDR_VDDQ
D8   GND   VDD_DDR_VDDQ   GND   VDD_DDR_VDDQ
D10   GND   VDD_PCIE_DIG_1P   GND   VDD_PCIE_DIG_1P
D12   GND   VDD_PCIE_1P8   GND   VDD_PCIE_1P8
D14   NC   NC   NC   NC
D16   GND   VDD_USB_3P3   GND   VDD_USB_3P3
D18   GND   VDD_USB_3P3   GND   VDD_USB_3P3
D20   GND   VDD_EMMC0_1P8_3   GND   VDD_EMMC0_1P8_3
D22   GND   VDD_EMMC0_VSELE   GND   VDD_EMMC0_VSELE
D24   GND   VDD_USDHC1_VSEL   GND   VDD_USDHC1_VSEL
D26   GND   VDD_USDHC1_1P8_   GND   VDD_USDHC1_1P8_
D28   GND   VDD_ENET0_1P8_2   GND   VDD_ENET0_1P8_2
D30   GND   VDD_ENET_MDIO_1   GND   VDD_ENET_MDIO_1
D32   GND   VDD_ESAI_SPDIF_   GND   VDD_ESAI_SPDIF_
D34   GND   VDD_ESAI_SPDIF_   GND   VDD_ESAI_SPDIF_
E1   GND   VDD_DDR_VDDQ   GND   VDD_DDR_VDDQ
E3   GND   VDD_DDR_VDDQ   GND   VDD_DDR_VDDQ
E5   GND   VDD_DDR_VDDQ   GND   VDD_DDR_VDDQ
E7   GND   VDD_DDR_VDDQ   GND   VDD_DDR_VDDQ
E9   GND   VDD_DDR_VDDQ   GND   VDD_DDR_VDDQ
E11   GND   VDD_PCIE_1P8   GND   VDD_PCIE_1P8
E13   NC   NC   NC   NC
E15   GND   NC   NC   NC
E17   GND   VDD_USB_3P3   GND   VDD_USB_3P3
E19   GND   VDD_USB_3P3   GND   VDD_USB_3P3
E21   GND   VDD_EMMC0_1P8_3   GND   VDD_EMMC0_1P8_3
E23   GND   VDD_USDHC1_VSEL   GND   VDD_USDHC1_VSEL
E25   GND   VDD_USDHC1_1P8_   GND   VDD_USDHC1_1P8_
E27   GND   VDD_ENET0_VSELE   GND   VDD_ENET0_VSELE
E29   GND   NC   NC   NC
E31   GND   VDD_ESAI_SPDIF_   GND   VDD_ESAI_SPDIF_
E33   GND   NC   NC   NC
E35   GND   VDD_ESAI_SPDIF_   GND   VDD_ESAI_SPDIF_
F2   GND   NC   NC   NC
F4   GND   NC   NC   NC
F6   GND   NC   NC   NC
F8   GND   NC   NC   NC
F10   GND   NC   NC   NC
F12   NC   NC   NC   NC
F14   GND   VDD_USB_3P3   GND   VDD_USB_3P3
F16   NC   NC   NC   NC
F18   GND   NC   NC   NC
F20   GND   NC   NC   NC
F22   GND   VDD_EMMC0_VSELE   GND   VDD_EMMC0_VSELE
F24   GND   NC   NC   NC
F26   GND   VDD_ENET0_VSELE   GND   VDD_ENET0_VSELE
F28   GND   VDD_ENET_MDIO_1   GND   VDD_ENET_MDIO_1
F30   GND   VDD_ESAI_SPDIF_   GND   VDD_ESAI_SPDIF_
F32   GND   VDD_ESAI_SPDIF_   GND   VDD_ESAI_SPDIF_
F34   GND   VDD_SPI_MCLK_UA   GND   VDD_SPI_MCLK_UA
G1   GND   VDD_DDR_VDDQ   GND   VDD_DDR_VDDQ
G3   GND   VDD_DDR_VDDQ   GND   VDD_DDR_VDDQ
G5   GND   VDD_DDR_VDDQ   GND   VDD_DDR_VDDQ
G7   GND   VDD_DDR_VDDQ   GND   VDD_DDR_VDDQ
G9   NC   NC   NC   NC
G11   PCIE0_PHY_PLL_R NC   NC   NC
G13   NC   VDD_PCIE_1P8   NC   NC
G15   GND   VDD_USB_3P3   GND   VDD_USB_3P3
G17   NC   NC   NC   NC
G19   GND   VDD_EMMC0_1P8_3   GND   VDD_EMMC0_1P8_3
G21   GND   VDD_EMMC0_VSELE   GND   VDD_EMMC0_VSELE
G23   GND   VDD_USDHC1_1P8_   GND   VDD_USDHC1_1P8_
G25   GND   VDD_ENET0_VSELE   GND   VDD_ENET0_VSELE
G27   GND   VDD_ENET0_1P8_2   GND   VDD_ENET0_1P8_2
G29   GND   VDD_ESAI_SPDIF_   GND   VDD_ESAI_SPDIF_
G31   GND   VDD_ESAI_SPDIF_   GND   VDD_ESAI_SPDIF_
G33   GND   VDD_SPI_MCLK_UA   GND   VDD_SPI_MCLK_UA
G35   GND   VDD_SPI_MCLK_UA   GND   VDD_SPI_MCLK_UA
H2   GND   VDD_DDR_VDDQ   GND   VDD_DDR_VDDQ
H4   GND   VDD_DDR_VDDQ   GND   VDD_DDR_VDDQ
H6   GND   VDD_DDR_VDDQ   GND   VDD_DDR_VDDQ
H8   GND   VDD_DDR_VDDQ   GND   VDD_DDR_VDDQ
H10   GND   VDD_PCIE_DIG_1P   GND   VDD_PCIE_DIG_1P
H12   NC   NC   NC   NC
H14   GND   VDD_USB_3P3   GND   VDD_USB_3P3
H16   NC   NC   NC   NC
H18   GND   VDD_USB_1P8   GND   VDD_USB_1P8
H20   GND   VDD_EMMC0_1P8_3   GND   VDD_EMMC0_1P8_3
H22   GND   VDD_EMMC0_VSELE   GND   VDD_EMMC0_VSELE
H24   GND   VDD_ENET0_VSELE   GND   VDD_ENET0_VSELE
H26   GND   VDD_ENET0_1P8_2   GND   VDD_ENET0_1P8_2
H28   GND   VDD_ESAI_SPDIF_   GND   VDD_ESAI_SPDIF_
H30   GND   NC   NC   NC
H32   GND   VDD_SPI_MCLK_UA   GND   VDD_SPI_MCLK_UA
H34   GND   VDD_SPI_MCLK_UA   GND   VDD_SPI_MCLK_UA
J1   GND   NC   NC   NC
J3   GND   NC   NC   NC
J5   GND   NC   NC   NC
J7   GND   NC   NC   NC
J9   GND   NC   NC   NC
J11   GND   NC   NC   NC
J13   GND   NC   NC   NC
J15   GND   NC   NC   NC
J17   GND   NC   NC   NC
J19   GND   NC   NC   NC
J21   GND   NC   NC   NC
J23   GND   NC   NC   NC
J25   GND   NC   NC   NC
J27   GND   NC   NC   NC
J29   GND   VDD_ESAI_SPDIF_   GND   VDD_ESAI_SPDIF_
J31   GND   VDD_SPI_MCLK_UA   GND   VDD_SPI_MCLK_UA
J33   GND   NC   NC   NC
J35   GND   VDD_SPI_SAI_1P8   GND   VDD_SPI_SAI_1P8
K2   GND   VDD_DDR_VDDQ   GND   VDD_DDR_VDDQ
K4   GND   VDD_DDR_VDDQ   GND   VDD_DDR_VDDQ
K6   GND   VDD_DDR_VDDQ   GND   VDD_DDR_VDDQ
K8   GND   VDD_DDR_VDDQ   GND   VDD_DDR_VDDQ
K10   GND   NC   NC   NC
K12   GND   NC   NC   NC
K14   GND   NC   NC   NC
K16   GND   NC   NC   NC
K18   GND   NC   NC   NC
K20   GND   NC   NC   NC
K22   GND   NC   NC   NC
K24   GND   NC   NC   NC
K26   GND   NC   NC   NC
K28   GND   VDD_ESAI_SPDIF_   GND   VDD_ESAI_SPDIF_
K30   GND   VDD_SPI_MCLK_UA   GND   VDD_SPI_MCLK_UA
K32   GND   VDD_SPI_MCLK_UA   GND   VDD_SPI_MCLK_UA
K34   GND   VDD_SPI_SAI_1P8   GND   VDD_SPI_SAI_1P8
L1   GND   VDD_DDR_VDDQ   GND   VDD_DDR_VDDQ
L3   GND   VDD_DDR_VDDQ   GND   VDD_DDR_VDDQ
L5   GND   VDD_DDR_VDDQ   GND   VDD_DDR_VDDQ
L7   GND   VDD_DDR_VDDQ   GND   VDD_DDR_VDDQ
L9   GND   NC   NC   NC
L11   NC   VDD_PCIE_DIG_1P   NC   NC
L13   NC   VDD_PCIE_LDO_1P   NC   NC
L15   NC   VDD_USB_3P3   NC   NC
L17   NC   VDD_USB_OTG_1P0   NC   NC
L19   NC   VDD_EMMC0_1P8_3   NC   NC
L21   NC   VDD_USDHC1_VSEL   NC   NC
L23   NC   VDD_ENET0_VSELE   NC   NC
L25   NC   VDD_ENET_MDIO_1   NC   NC
L27   GND   NC   NC   NC
L29   GND   VDD_SPI_MCLK_UA   GND   VDD_SPI_MCLK_UA
L31   GND   VDD_SPI_MCLK_UA   GND   VDD_SPI_MCLK_UA
L33   GND   VDD_SPI_SAI_1P8   GND   VDD_SPI_SAI_1P8
L35   GND   VDD_SPI_SAI_1P8   GND   VDD_SPI_SAI_1P8
M2   GND   NC   NC   NC
M4   GND   NC   NC   NC
M6   GND   NC   NC   NC
M8   GND   NC   NC   NC
M10   GND   NC   NC   NC
M12   NC   VDD_DDR_VDDQ   NC   NC
M14   NC   VDD_ANA0_1P8   NC   NC
M16   NC   VDD_USB_SS3_LDO   NC   NC
M18   NC   VDD_USB_1P8   NC   NC
M20   NC   VDD_EMMC0_VSELE   NC   NC
M22   NC   VDD_USDHC1_1P8_   NC   NC
M24   NC   VDD_ENET0_1P8_2   NC   NC
M26   GND   NC   NC   NC
M28   GND   VDD_SPI_MCLK_UA   GND   VDD_SPI_MCLK_UA
M30   GND   NC   NC   NC
M32   GND   VDD_SPI_SAI_1P8   GND   VDD_SPI_SAI_1P8
M34   GND   VDD_SPI_SAI_1P8   GND   VDD_SPI_SAI_1P8
N1   GND   VDD_DDR_VDDQ   GND   VDD_DDR_VDDQ
N3   GND   VDD_DDR_VDDQ   GND   VDD_DDR_VDDQ
N5   GND   VDD_DDR_VDDQ   GND   VDD_DDR_VDDQ
N7   GND   VDD_DDR_VDDQ   GND   VDD_DDR_VDDQ
N9   NC   VDD_DDR_VDDQ   NC   NC
N11   NC   VDD_DDR_VDDQ   NC   NC
N13   GND   NC   NC   NC
N15   NC   VDD_MAIN   NC   NC
N17   GND   NC   NC   NC
N19   NC   VDD_MAIN   NC   NC
N21   GND   NC   NC   NC
N23   NC   VDD_GPU   NC   NC
N25   NC   VDD_ESAI_SPDIF_   NC   NC
N27   GND   NC   NC   NC
N29   GND   VDD_SPI_MCLK_UA   GND   VDD_SPI_MCLK_UA
N31   GND   VDD_SPI_SAI_1P8   GND   VDD_SPI_SAI_1P8
N33   GND   NC   NC   NC
N35   GND   VDD_SPI_SAI_1P8   GND   VDD_SPI_SAI_1P8
P2   GND   VDD_DDR_VDDQ   GND   VDD_DDR_VDDQ
P4   GND   VDD_DDR_VDDQ   GND   VDD_DDR_VDDQ
P6   GND   VDD_DDR_VDDQ   GND   VDD_DDR_VDDQ
P8   GND   VDD_DDR_VDDQ   GND   VDD_DDR_VDDQ
P10   GND   NC   NC   NC
P12   NC   VDD_MAIN   NC   NC
P14   GND   NC   NC   NC
P16   NC   VDD_MAIN   NC   NC
P18   GND   NC   NC   NC
P20   NC   VDD_GPU   NC   NC
P22   NC   VDD_GPU   NC   NC
P24   NC   VDD_MAIN   NC   NC
P26   GND   NC   NC   NC
P28   GND   VDD_SPI_SAI_1P8   GND   VDD_SPI_SAI_1P8
P30   GND   VDD_SPI_SAI_1P8   GND   VDD_SPI_SAI_1P8
P32   GND   VDD_SPI_SAI_1P8   GND   VDD_SPI_SAI_1P8
P34   GND   VDD_SPI_SAI_1P8   GND   VDD_SPI_SAI_1P8
R1   GND   NC   NC   NC
R3   GND   NC   NC   NC
R5   GND   NC   NC   NC
R7   NC   VDD_DDR_VDDQ   NC   NC
R9   GND   NC   NC   NC
R11   NC   VDD_DDR_VDDQ   NC   NC
R13   NC   VDD_MAIN   NC   NC
R15   GND   NC   NC   NC
R17   NC   VDD_MAIN   NC   NC
R19   GND   NC   NC   NC
R21   NC   VDD_GPU   NC   NC
R23   GND   NC   NC   NC
R25   NC   VDD_SPI_MCLK_UA   NC   NC
R27   GND   NC   NC   NC
R29   GND   VDD_SPI_SAI_1P8   GND   VDD_SPI_SAI_1P8
R31   GND   VDD_SPI_SAI_1P8   GND   VDD_SPI_SAI_1P8
R33   GND   VDD_SPI_SAI_1P8   GND   VDD_SPI_SAI_1P8
R35   GND   VDD_SPI_SAI_1P8   GND   VDD_SPI_SAI_1P8
T2   GND   VDD_DDR_VDDQ   GND   VDD_DDR_VDDQ
T4   GND   VDD_DDR_VDDQ   GND   VDD_DDR_VDDQ
T6   GND   VDD_DDR_VDDQ   GND   VDD_DDR_VDDQ
T8   GND   VDD_DDR_VDDQ   GND   VDD_DDR_VDDQ
T10   GND   NC   NC   NC
T12   NC   VDD_DDR_VDDQ   NC   NC
T14   NC   VDD_MAIN   NC   NC
T16   GND   NC   NC   NC
T18   NC   VDD_MAIN   NC   NC
T20   GND   NC   NC   NC
T22   NC   VDD_GPU   NC   NC
T24   GND   NC   NC   NC
T26   GND   NC   NC   NC
T28   GND   NC   NC   NC
T30   GND   NC   NC   NC
T32   GND   NC   NC   NC
T34   GND   NC   NC   NC
U1   GND   VDD_DDR_VDDQ   GND   VDD_DDR_VDDQ
U3   GND   VDD_DDR_VDDQ   GND   VDD_DDR_VDDQ
U5   GND   VDD_DDR_VDDQ   GND   VDD_DDR_VDDQ
U7   GND   VDD_DDR_VDDQ   GND   VDD_DDR_VDDQ
U9   GND   NC   NC   NC
U11   NC   VDD_DDR_VDDQ   NC   NC
U13   GND   NC   NC   NC
U15   NC   VDD_MAIN   NC   NC
U17   GND   NC   NC   NC
U19   NC   VDD_MAIN   NC   NC
U21   GND   NC   NC   NC
U23   NC   VDD_GPU   NC   NC
U25   NC   VDD_SPI_SAI_1P8   NC   NC
U27   GND   NC   NC   NC
U29   NC   ADC_VREFH   NC   NC
U31   ADC_VREFL   NC   NC   NC
U33   GND   VDD_ADC_DIG_1P8   GND   VDD_ADC_DIG_1P8
U35   GND   VDD_ADC_DIG_1P8   GND   VDD_ADC_DIG_1P8
V2   GND   NC   NC   NC
V4   GND   NC   NC   NC
V6   GND   NC   NC   NC
V8   GND   NC   NC   NC
V10   GND   NC   NC   NC
V12   NC   VDD_MAIN   NC   NC
V14   GND   NC   NC   NC
V16   NC   VDD_MAIN   NC   NC
V18   GND   NC   NC   NC
V20   NC   VDD_GPU   NC   NC
V22   GND   NC   NC   NC
V24   NC   VDD_MAIN   NC   NC
V26   GND   NC   NC   NC
V28   NC   VDD_ADC_1P8   NC   NC
V30   GND   VDD_ADC_DIG_1P8   GND   VDD_ADC_DIG_1P8
V32   GND   VDD_ADC_DIG_1P8   GND   VDD_ADC_DIG_1P8
V34   GND   VDD_ADC_DIG_1P8   GND   VDD_ADC_DIG_1P8
W1   GND   VDD_DDR_VDDQ   GND   VDD_DDR_VDDQ
W3   GND   VDD_DDR_VDDQ   GND   VDD_DDR_VDDQ
W5   GND   VDD_DDR_VDDQ   GND   VDD_DDR_VDDQ
W7   GND   VDD_DDR_VDDQ   GND   VDD_DDR_VDDQ
W9   GND   NC   NC   NC
W11   NC   VDD_DDR_VDDQ   NC   NC
W13   NC   VDD_MAIN   NC   NC
W15   GND   NC   NC   NC
W17   NC   VDD_MAIN   NC   NC
W19   GND   NC   NC   NC
W21   NC   VDD_GPU   NC   NC
W23   GND   NC   NC   NC
W25   NC   VDD_ADC_DIG_1P8   NC   NC
W27   GND   NC   NC   NC
W29   GND   VDD_ADC_DIG_1P8   GND   VDD_ADC_DIG_1P8
W31   GND   NC   NC   NC
W33   GND   NC   NC   NC
W35   GND   NC   NC   NC
Y2   GND   VDD_DDR_VDDQ   GND   VDD_DDR_VDDQ
Y4   GND   VDD_DDR_VDDQ   GND   VDD_DDR_VDDQ
Y6   GND   VDD_DDR_VDDQ   GND   VDD_DDR_VDDQ
Y8   GND   VDD_DDR_VDDQ   GND   VDD_DDR_VDDQ
Y10   GND   NC   NC   NC
Y12   NC   VDD_DDR_VDDQ   NC   NC
Y14   NC   VDD_MAIN   NC   NC
Y16   GND   NC   NC   NC
Y18   NC   VDD_MAIN   NC   NC
Y20   GND   NC   NC   NC
Y22   NC   VDD_MAIN   NC   NC
Y24   NC   VDD_CAN_UART_1P   NC   NC
Y26   GND   NC   NC   NC
Y28   GND   NC   NC   NC
Y30   GND   NC   NC   NC
Y32   GND   VDD_CAN_UART_1P   GND   VDD_CAN_UART_1P
Y34   GND   VDD_CAN_UART_1P   GND   VDD_CAN_UART_1P
AA1   GND   NC   NC   NC
AA3   GND   NC   NC   NC
AA5   GND   NC   NC   NC
AA7   GND   NC   NC   NC
AA9   NC   VDD_DDR_VDDQ   NC   NC
AA11   NC   VDD_DDR_VDDQ   NC   NC
AA13   GND   NC   NC   NC
AA15   NC   VDD_A35   NC   NC
AA17   NC   VDD_A35   NC   NC
AA19   NC   VDD_A35   NC   NC
AA21   GND   NC   NC   NC
AA23   NC   VDD_MAIN   NC   NC
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| Models and submodels in the file (93): BDPROGSCARUDQP_SDMMC_3V3SF_00 (I/O), BDPROGSCARUDQP_SDMMC_3V3SF_01 (I/O), BDPROGSCARUDQP_SDMMC_3V3SF_10_2v7 (I/O), BDPROGSCARUDQP_SDMMC_3V3SF_10 (I/O), BDPROGSCARUDQP_SDMMC_3V3SF_11_2v7 (I/O), BDPROGSCARUDQP_SDMMC_3V3SF_11 (I/O), BD_1mA (I/O), BD_2mA (I/O), BD_4mA (I/O), BD_6mA (I/O), BD_8mA (I/O), BD_10mA (I/O), BD_12mA (I/O), BD_HS (I/O), DWC_D5MCK3L_34 (I/O), DWC_D5MCK3L_40 (I/O), DWC_D5MCK3L_48 (I/O), DWC_D5MCKL4_40 (I/O), DWC_D5MCKL4_48 (I/O), DWC_D5MCKL4_60 (I/O), DWC_D5MCKL4_80 (I/O), DWC_D5MC3L_34 (I/O), DWC_D5MC3L_40 (I/O), DWC_D5MC3L_48 (I/O), DWC_D5MCL4_40 (I/O), DWC_D5MCL4_48 (I/O), DWC_D5MCL4_60 (I/O), DWC_D5MCL4_80 (I/O), DWC_D5MP3L_34 (I/O), DWC_D5MP3L_40 (I/O), DWC_D5MP3L_48 (I/O), DWC_D5MP3L_ODT40 (Input), DWC_D5MP3L_ODT60 (Input), DWC_D5MP3L_ODTOFF (Input), DWC_D5MPL4_40 (I/O), DWC_D5MPL4_48 (I/O), DWC_D5MPL4_60 (I/O), DWC_D5MPL4_80 (I/O), DWC_D5MPL4_ODT40 (Input), DWC_D5MPL4_ODT48 (Input), DWC_D5MPL4_ODT60 (Input), DWC_D5MPL4_ODT80 (Input), DWC_D5MPL4_ODTOFF (Input), DWC_D5MPD3L_34 (I/O), DWC_D5MPD3L_40 (I/O), DWC_D5MPD3L_48 (I/O), DWC_D5MPD3L_ODT40 (Input), DWC_D5MPD3L_ODT60 (Input), DWC_D5MPD3L_ODTOFF (Input), DWC_D5MPDL4_40 (I/O), DWC_D5MPDL4_48 (I/O), DWC_D5MPDL4_60 (I/O), DWC_D5MPDL4_80 (I/O), DWC_D5MPDL4_ODT40 (Input), DWC_D5MPDL4_ODT48 (Input), DWC_D5MPDL4_ODT60 (Input), DWC_D5MPDL4_ODT80 (Input), DWC_D5MPDL4_ODTOFF (Input), MIPI_HS_CSI (Input), MIPI_LP_CSI (Input), LVDS_TX (3-state), MIPI_HS_DSI (Output), MIPI_LP_DSI (I/O), BDPROG_00 (I/O), BDPROG_01 (I/O), BDPROG_10 (I/O), BDPROG_11 (I/O), abi_in (Input), abi_out (Output), RGMII_RX_2V5_mi (Input), RGMII_TX_2V5_drv0_mo (3-state), RGMII_TX_2V5_drv1_mo (3-state), hs_input (Input), hs_ls_input (Input), hs_vbus_input (Input), hsfs_host_input (Input), hsfs_device_dp_input (Input), hsfs_device_dm_input (Input), hs_driver (Output), hs_fs_driver (Output)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
